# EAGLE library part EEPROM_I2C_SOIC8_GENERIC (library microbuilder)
Note: The same pinout is used for many I2C EEPROMs in SOIC8(150mil) from a variety of manufacturers and in various sizes. Examples: 16K (2K x 8 Bit) I2C EEPROM 1.7-5.5V, 400KHz, -40°C-85°C Digikey: CAT24C16WI-GT3CT-ND 256K (32K x 8 Bit) I2C EEPROM 1.7-5.5V, 400KHz, -40°C-85°C Digikey: 24AA256-I/SN-ND
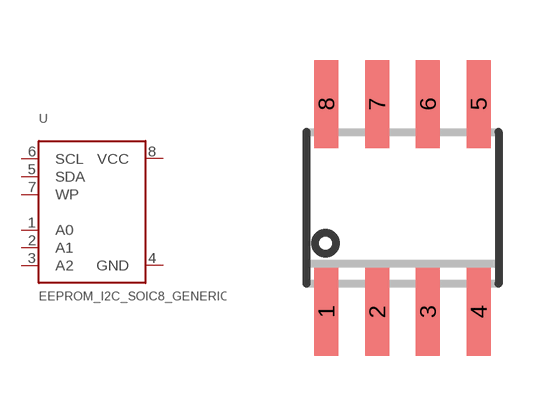
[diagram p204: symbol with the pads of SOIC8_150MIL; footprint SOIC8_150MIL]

Designator prefix U

## EEPROM_I2C_SOIC8_GENERIC  [SOIC8_150MIL]
1  A0  in
2  A1  in
3  A2  in
4  GND  pwr
5  SDA
6  SCL  in
7  WP  in
8  VCC  pwr

## Footprint SOIC8_150MIL (pad centres in mm)
Small Outline IC - 150mil Wide
smd 0.6 x 2.2: 1 -1.905,-2.6; 2 -0.635,-2.6; 3 0.635,-2.6; 4 1.905,-2.6; 5 1.905,2.6; 6 0.635,2.6; 7 -0.635,2.6; 8 -1.905,2.6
